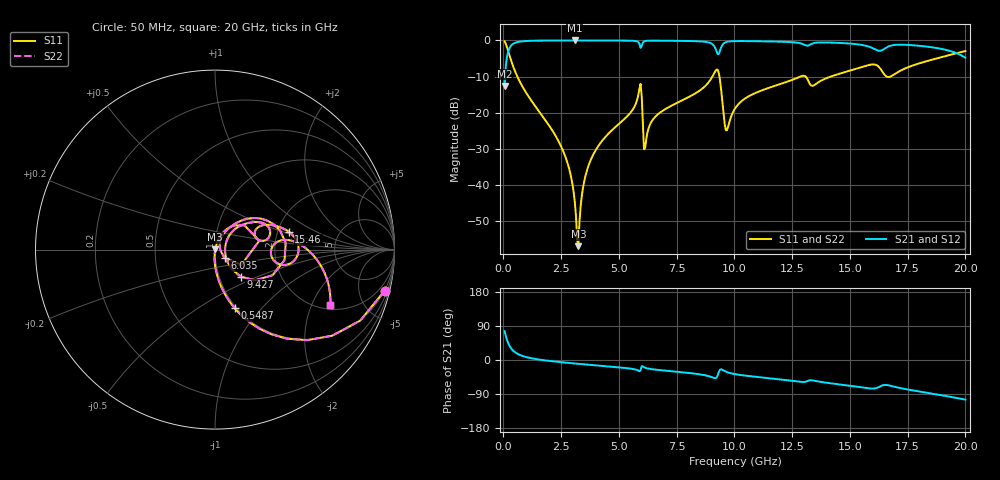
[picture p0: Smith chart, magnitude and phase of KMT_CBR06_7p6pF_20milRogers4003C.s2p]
! Data measured by Modelithics Inc. support@modelithics.com 813-866-6335
! KEMET CBR0603 7.6pF, Pad Width= 0.851mm, Pad Length= 0.64mm, Pad Gap= 0.62mm, 20mil Rogers 4003C substrate Data, January 2022
# hz S ma R 50
! 2 Port Network Data from SP1.SP block
! freq  magS11  angS11  magS21  angS21  magS12  angS12  magS22  angS22
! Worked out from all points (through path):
!   401 points, 50 MHz to 20 GHz, reference 50 ohm
!   highest |S21| = -0.01 dB at 3.092 GHz (marker M1); lowest = -12.6 dB at 50 MHz (marker M2)
!   group delay of S21, straight-line fit = 14.9 ps
!   lowest |S11| = -56.9 dB at 3.242 GHz (marker M3), VSWR 1.00, Z = 50.1 + j0.0579 ohm
!   |S11| at or under -10 dB: 601.9 MHz to 9.046 GHz (8.444 GHz wide, 175 % of centre); 9.35 GHz to 12.85 GHz (3.503 GHz wide, 31.5 % of centre); 13.08 GHz to 14.17 GHz (1.086 GHz wide, 7.97 % of centre)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
!   |S22| runs from -56.9 to -0.2 dB; largest |S21 - S12| = 0
!   S11 on the Smith chart (normalised r, x): 50 MHz: 0.98, -8.21; 548.8 MHz: 0.98, -0.73; 6.035 GHz: 1.11, -0.10; 9.427 GHz: 1.26, -0.40; 15.46 GHz: 2.30, +0.56; 20 GHz: 2.21, -2.76
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5e7  0.9721 -13.7  0.2341 76.3  0.2341 76.3  0.9721 -13.7
2.495e8  0.6372 -51.1  0.7699 38.8  0.7699 38.8  0.6372 -51.1
5.4875e8  0.3451 -71.4  0.9378 18.5  0.9378 18.5  0.3451 -71.4
2.54375e9  0.03173 -94.2  0.9983 -6.1  0.9983 -6.1  0.03173 -94.2
2.892875e9  0.01457 -93.7  0.9987 -8.1  0.9987 -8.1  0.01457 -93.7
3.092375e9  0.005709 -87.6  0.9987 -9.3  0.9987 -9.3  0.005709 -87.6
3.242e9  0.00143 23.8  0.9987 -10.1  0.9987 -10.1  0.00143 23.8
3.391625e9  0.007074 69.2  0.9986 -10.9  0.9986 -10.9  0.007074 69.2
3.94025e9  0.0284 73.5  0.9981 -13.8  0.9981 -13.8  0.0284 73.5
5.8355e9  0.174 51.1  0.9516 -27.9  0.9516 -27.9  0.174 51.1
6.035e9  0.07068 -41.3  0.9349 -17.0  0.9349 -17.0  0.07068 -41.3
6.184625e9  0.0436 52.1  0.9866 -21.5  0.9866 -21.5  0.0436 52.1
6.73325e9  0.09792 61.8  0.9918 -26.4  0.9918 -26.4  0.09792 61.8
9.177125e9  0.3779 16.2  0.7762 -48.1  0.7762 -48.1  0.3779 16.2
9.4265e9  0.2069 -46.4  0.8048 -24.5  0.8048 -24.5  0.2069 -46.4
9.675875e9  0.05728 8.9  0.9556 -31.8  0.9556 -31.8  0.05728 8.9
1.0025e10  0.1142 45.0  0.9778 -37.2  0.9778 -37.2  0.1142 45.0
1.286788e10  0.3176 25.5  0.9103 -57.6  0.9103 -57.6  0.3176 25.5
1.336662e10  0.2352 18.7  0.9028 -53.7  0.9028 -53.7  0.2352 18.7
1.546138e10  0.4232 13.6  0.8725 -71.9  0.8725 -71.9  0.4232 13.6
1.670825e10  0.313 -0.3  0.8347 -67.3  0.8347 -67.3  0.313 -0.3
2e10  0.7123 -25.6  0.5768 -104.5  0.5768 -104.5  0.7123 -25.6
